(* Logix 5000 Rung export; software revision 16.04 *)

TYPE RLX2_UTIL :   // Internal tag used for internal ladder processing. Not to be updated by user application
STRUCT
   ImgVersionInformation : SINT[28];   // *Do Not Modify*
   RadioInformation : SINT[296];   // *Do Not Modify*
   CRCInformation : DINT[20];   // *Do Not Modify*
   TotalupTime : DINT;   // *Do Not Modify*
   TotalLinkTime : DINT;   // *Do Not Modify*
END_STRUCT
END_TYPE

TYPE RLX2_CONTROL :   // Contains trigger bit for the functions supported by the RLX2. Bit should be set as 1 to trigger AOI request
STRUCT
   GetStatusData : BOOL;   // Reads Diagnostic status data from RLX2
   GetCRCSignature : BOOL;   // Read CRC File Signature Information
END_STRUCT
END_TYPE

TYPE RLX2_STATUS :   // RLX2 Radio Status Data
STRUCT
   SSID : SINT[32];   // The Service Set Identifier is a name assigned to the wireless network
   IPAddress : INT[4];   // Radio's IP address
   MACAddress : SINT[6];   // Physical Media Access Control (MAC) address of the device
   NetworkMode : SINT;   // RLX2 radio Network mode (Master= 6 Repeater=7 Client=1)
   ConnectionState : SINT;   // Connection State of Radio
   SignalStrength : INT;   // Current Strength of the signal in dBm
   Channel : INT;   // Current Channel in which RLX2 is transmitting
   WEP : SINT;   // WEP encryption key
   Flags : DINT;   // Flags: Flag[0/1]= Extension channel Flag[2]= SSIDhidden Flag[3]=Allow Children Flag[4/5]=STP/RSTP Flag[6]=TXusingGI
   MasterMACAddress : SINT[6];   // MAC Address of Parent Radio in which Repeater or Client is linked
   HopCount : SINT;   // Number of hops to the master
   PortStatus : SINT;   // Ethernet Port Status (Speed 1=10Mb/s 2=100Mb/s 3=1000Mb/s)
   Associations : INT;   // Number of network elements to which radio has wireless connection
   BridgeAssociations : INT;   // Number of devices to which radio has wireless connection
   TxRadioThroughput : DINT;   // Transmit throughput in kilobits per second
   RxRadioThroughput : DINT;   // Receive throughput in kilobits per second
   Uptime : RLX2_UPTIME;   // This is the amount of time the radio has been running since power up (Days/Hours/Minutes/Seconds)
   LinkTime : RLX2_LINKTIME;   // The time the radio has been linked (Days/Hours/Minutes/Seconds)
   TxPacketRate : DINT;   // Total number of packets transmitted
   RxPacketRate : DINT;   // Total number of packets received
   ModuleName : SINT[32];   // The name of the radio
   ProductName : SINT[32];   // Name of product family
   ImageVerStr : SINT[28];   // Firmware version loaded in device
   TxGood : DINT;   // Number of Good Transmitted Frames
   RxGood : DINT;   // Number of Good Received Frames
   TxBad : DINT;   // Number of Bad Transmitted Frames
   RxBad : DINT;   // Number of Bad Received Frames
   TxDirectedFrames : DINT;   // Number of Transmitted Directed Frames
   TxMulticastFrames : DINT;   // Number of Transmitted Multicast Frames
   TxBroadcastFrames : DINT;   // Number of Transmitted Broadcast Frames
   RxDirectedFrames : DINT;   // Number of Received Directed Frames
   RxMulticastFrames : DINT;   // Number of Received Multicast Frames
   RxBroadcastFrames : DINT;   // Number of Received Broadcast Frames
   RxCRCErr : DINT;   // Number of CRC Errors
   Retries : SINT;   // Percentage retransmission (0-100%)
   Utilization : SINT;   // Measured channel utilization (0-100%)
   ChannelWidth : SINT;   // Configured channel width (20 or 40 MHz)
   Antennas : SINT;   // Active Antenna Information
   TxRate : INT;   // Encoded Current Tx Rate to Parent (Client/Repeater Only)
   TxBitRate : INT;   // Actual Tx Bit Rate to Parent in 100 kb/s units
   TxBcastRate : INT;   // Broadcast packet rate being sent to radio (pps)
   TxMcstRate : INT;   // Multicast packet rate being sent to radio (pps)
   Reserved1 : DINT;   // Reserved
   Reserved2 : DINT;   // Reserved
   Reserved3 : DINT;   // Reserved
   Reserved4 : DINT;   // Reserved
   Reserved5 : DINT;   // Reserved
   Reserved6 : DINT;   // Reserved
   Reserved7 : DINT;   // Reserved
   Reserved8 : DINT;   // Reserved
   Reserved9 : DINT;   // Reserved
   Reserved10 : DINT;   // Reserved
   Reserved11 : DINT;   // Reserved
   Reserved12 : DINT;   // Reserved
   Reserved13 : DINT;   // Reserved
   Reserved14 : DINT;   // Reserved
   Reserved15 : DINT;   // Reserved
   Reserved16 : DINT;   // Reserved
END_STRUCT
END_TYPE

TYPE RLX2_LINKTIME :   // RLX2 Repeater Link Time
STRUCT
   Days : DINT;   // Number of Days Repeater has been connected with a Master
   Hours : DINT;   // Number of Hours Repeater has been connected with a Master
   Minutes : DINT;   // Number of Minutes Repeater has been connected with a Master
   Seconds : DINT;   // Number of Seconds Repeater has been connected with a Master
END_STRUCT
END_TYPE

TYPE RLX2_UPTIME :
STRUCT
   Days : DINT;
   Hours : DINT;
   Minutes : DINT;
   Seconds : DINT;
END_STRUCT
END_TYPE

TYPE RLX2_CRC :   // CRC File Signature Information
STRUCT
   OS_Sig : DINT;   // CRC signature of OS related files
   Wireless_Sig : DINT;   // CRC signature of Wireless related files
   Config_Sig : DINT;   // CRC signature of Configuration related files
   Security_Sig : DINT;   // CRC signature of Security related files
   Web_Sig : DINT;   // CRC signature of the web pages image file.
   SDCard_Sig : DINT;   // CRC signature of the contents of the SD Card
   Reserved1 : DINT;   // Reserved
   Reserved2 : DINT;   // Reserved
   Reserved3 : DINT;   // Reserved
   Reserved4 : DINT;   // Reserved
   Reserved5 : DINT;   // Reserved
   Reserved6 : DINT;   // Reserved
   Reserved7 : DINT;   // Reserved
   Reserved8 : DINT;   // Reserved
   Reserved9 : DINT;   // Reserved
   Reserved10 : DINT;   // Reserved
   Reserved11 : DINT;   // Reserved
   Reserved12 : DINT;   // Reserved
   Reserved13 : DINT;   // Reserved
   Reserved14 : DINT;   // Reserved
END_STRUCT
END_TYPE

TYPE RLX2_ModuleDef :   // Main RLX2 Radio definition
STRUCT
   CONTROL : RLX2_CONTROL;   // Trigger bits used to request functions from RLX2 Radio
   STATUS : RLX2_STATUS;   // RLX2 radio diagnostic data
   CRC : RLX2_CRC;   // RLX2 CRC file signature Information
   UTIL : RLX2_UTIL;   // *Do Not Modify*
END_STRUCT
END_TYPE

ADD_ON_INSTRUCTION AOI_RLX2   (* revision 2.0, vendor ProSoft Technology Inc., ExecutePrescan *)
// Add-On Instruction for RLX2 Industrial Hotspot
// Revision note:
// 2.0 -- Added Support for Extended Status and CRC File Information (v38)
// Help:
// 1.5 - Fix to Logic to display correct RSSI
// 1.4 --  Change the display information for the Link and Uptime of the radio
VAR_IN_OUT
   RLX2 : RLX2_ModuleDef; {required}
   RLX2_MSG_GET_IMG_VER : MESSAGE; {required}
   RLX2_MSG_GET_STATUS : MESSAGE; {required}
   RLX2_MSG_GET_CRC_SIG : MESSAGE; {required}
END_VAR
VAR
   Hold64 : INT[2];
   HoldRSSI : INT;
   Hold66 : INT[2];
   ImgVersion : DINT;
   TriggerStatusMSG : BOOL;   // Trigger Status Information MSG
END_VAR

ROUTINE Logic   (* ladder *)
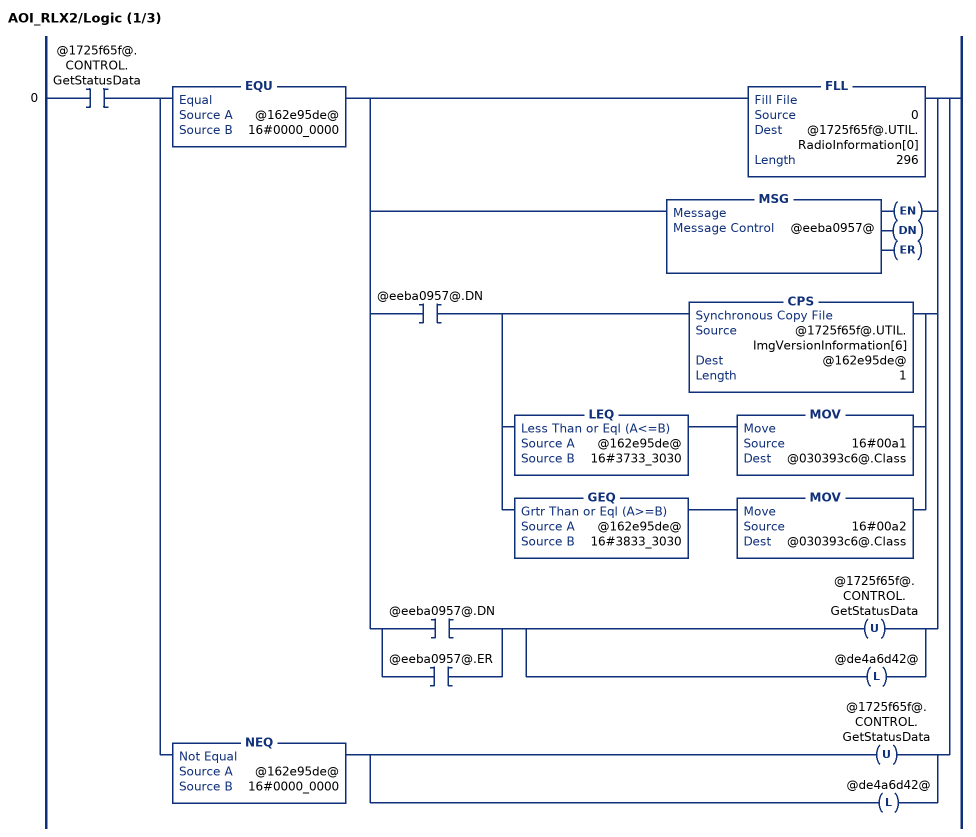
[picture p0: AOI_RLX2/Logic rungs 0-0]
   0: XIC(@1725f65f@.CONTROL.GetStatusData)[EQU(@162e95de@,16#0000_0000) [FLL(0,@1725f65f@.UTIL.RadioInformation[0],296) ,MSG(@eeba0957@) ,[XIC(@eeba0957@.DN) [CPS(@1725f65f@.UTIL.ImgVersionInformation[6],@162e95de@,1) ,LEQ(@162e95de@,16#3733_3030) MOV(16#00a1,@030393c6@.Class) ,GEQ(@162e95de@,16#3833_3030) MOV(16#00a2,@030393c6@.Class) ] ,[XIC(@eeba0957@.DN) ,XIC(@eeba0957@.ER) ] [OTU(@1725f65f@.CONTROL.GetStatusData) ,OTL(@de4a6d42@) ] ] ] ,NEQ(@162e95de@,16#0000_0000) [OTU(@1725f65f@.CONTROL.GetStatusData) ,OTL(@de4a6d42@) ] ];
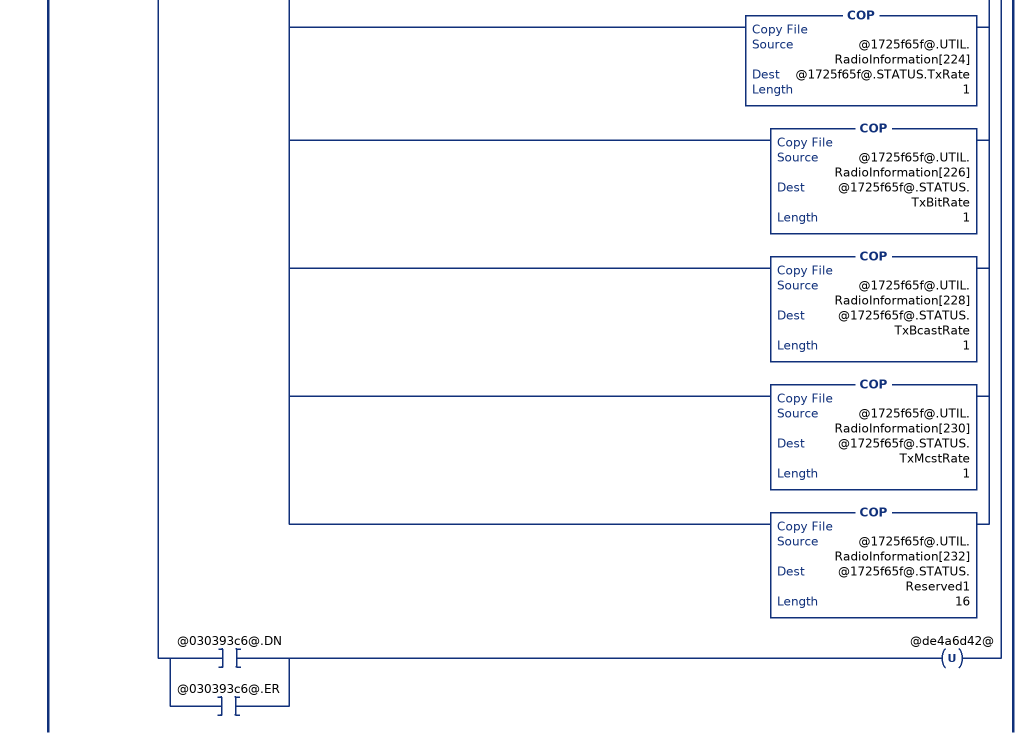
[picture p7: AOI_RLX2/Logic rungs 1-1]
   1: XIC(@de4a6d42@)[MSG(@030393c6@) ,[XIC(@030393c6@.DN) [COP(@1725f65f@.UTIL.RadioInformation[0],@1725f65f@.STATUS.SSID[0],32) ,MVM(@1725f65f@.UTIL.RadioInformation[32],255,@1725f65f@.STATUS.IPAddress[0]) ,MVM(@1725f65f@.UTIL.RadioInformation[33],255,@1725f65f@.STATUS.IPAddress[1]) ,MVM(@1725f65f@.UTIL.RadioInformation[34],255,@1725f65f@.STATUS.IPAddress[2]) ,MVM(@1725f65f@.UTIL.RadioInformation[35],255,@1725f65f@.STATUS.IPAddress[3]) ,COP(@1725f65f@.UTIL.RadioInformation[36],@1725f65f@.STATUS.MACAddress[0],6) ,COP(@1725f65f@.UTIL.RadioInformation[42],@1725f65f@.STATUS.NetworkMode,1) ,COP(@1725f65f@.UTIL.RadioInformation[43],@1725f65f@.STATUS.ConnectionState,1) ,NEQ(@1725f65f@.STATUS.NetworkMode,6) COP(@1725f65f@.UTIL.RadioInformation[44],@0dfc57aa@,1) SUB(@0dfc57aa@,100,@1725f65f@.STATUS.SignalStrength) ,MVM(@1725f65f@.UTIL.RadioInformation[46],255,@1725f65f@.STATUS.Channel) ,COP(@1725f65f@.UTIL.RadioInformation[47],@1725f65f@.STATUS.WEP,1) ,COP(@1725f65f@.UTIL.RadioInformation[48],@1725f65f@.STATUS.Flags,4) ,COP(@1725f65f@.UTIL.RadioInformation[52],@1725f65f@.STATUS.MasterMACAddress[0],6) ,COP(@1725f65f@.UTIL.RadioInformation[58],@1725f65f@.STATUS.HopCount,1) ,COP(@1725f65f@.UTIL.RadioInformation[59],@1725f65f@.STATUS.PortStatus,1) ,COP(@1725f65f@.UTIL.RadioInformation[60],@1725f65f@.STATUS.Associations,2) ,COP(@1725f65f@.UTIL.RadioInformation[62],@1725f65f@.STATUS.BridgeAssociations,2) ,COP(@1725f65f@.UTIL.RadioInformation[64],@dc9c6250@[0],1) COP(@dc9c6250@[0],@1725f65f@.STATUS.TxRadioThroughput,1) ,COP(@1725f65f@.UTIL.RadioInformation[66],@0cd69a93@[0],1) COP(@0cd69a93@[0],@1725f65f@.STATUS.RxRadioThroughput,1) ,[COP(@1725f65f@.UTIL.RadioInformation[68],@1725f65f@.UTIL.TotalupTime,4) ,CPT(@1725f65f@.STATUS.Uptime.Days,(@1725f65f@.UTIL.TotalupTime/60/60/24)) ,CPT(@1725f65f@.STATUS.Uptime.Hours,(@1725f65f@.UTIL.TotalupTime/60/60)-(@1725f65f@.STATUS.Uptime.Days*24)) ,CPT(@1725f65f@.STATUS.Uptime.Minutes,(@1725f65f@.UTIL.TotalupTime/60)-(@1725f65f@.STATUS.Uptime.Days*24*60)-(@1725f65f@.STATUS.Uptime.Hours*60)) ,CPT(@1725f65f@.STATUS.Uptime.Seconds,(@1725f65f@.UTIL.TotalupTime)-(@1725f65f@.STATUS.Uptime.Days*24*60*60)-(@1725f65f@.STATUS.Uptime.Hours*60*60)-(@1725f65f@.STATUS.Uptime.Minutes*60)) ] ,[COP(@1725f65f@.UTIL.RadioInformation[72],@1725f65f@.UTIL.TotalLinkTime,4) ,CPT(@1725f65f@.STATUS.LinkTime.Days,(@1725f65f@.UTIL.TotalLinkTime/60/60/24)) ,CPT(@1725f65f@.STATUS.LinkTime.Hours,(@1725f65f@.UTIL.TotalLinkTime/60/60)-(@1725f65f@.STATUS.LinkTime.Days*24)) ,CPT(@1725f65f@.STATUS.LinkTime.Minutes,(@1725f65f@.UTIL.TotalLinkTime/60)-(@1725f65f@.STATUS.LinkTime.Days*24*60)-(@1725f65f@.STATUS.LinkTime.Hours*60)) ,CPT(@1725f65f@.STATUS.LinkTime.Seconds,(@1725f65f@.UTIL.TotalLinkTime)-(@1725f65f@.STATUS.LinkTime.Days*24*60*60)-(@1725f65f@.STATUS.LinkTime.Hours*60*60)-(@1725f65f@.STATUS.LinkTime.Minutes*60)) ] ,COP(@1725f65f@.UTIL.RadioInformation[76],@1725f65f@.STATUS.TxPacketRate,4) ,COP(@1725f65f@.UTIL.RadioInformation[80],@1725f65f@.STATUS.RxPacketRate,4) ,COP(@1725f65f@.UTIL.RadioInformation[84],@1725f65f@.STATUS.ModuleName[0],32) ,COP(@1725f65f@.UTIL.RadioInformation[116],@1725f65f@.STATUS.ProductName[0],32) ,COP(@1725f65f@.UTIL.RadioInformation[148],@1725f65f@.STATUS.ImageVerStr[0],28) ,COP(@1725f65f@.UTIL.RadioInformation[176],@1725f65f@.STATUS.TxGood,4) ,COP(@1725f65f@.UTIL.RadioInformation[180],@1725f65f@.STATUS.RxGood,4) ,COP(@1725f65f@.UTIL.RadioInformation[184],@1725f65f@.STATUS.TxBad,4) ,COP(@1725f65f@.UTIL.RadioInformation[188],@1725f65f@.STATUS.RxBad,4) ,COP(@1725f65f@.UTIL.RadioInformation[192],@1725f65f@.STATUS.TxDirectedFrames,4) ,COP(@1725f65f@.UTIL.RadioInformation[196],@1725f65f@.STATUS.TxMulticastFrames,4) ,COP(@1725f65f@.UTIL.RadioInformation[200],@1725f65f@.STATUS.TxBroadcastFrames,4) ,COP(@1725f65f@.UTIL.RadioInformation[204],@1725f65f@.STATUS.RxDirectedFrames,4) ,COP(@1725f65f@.UTIL.RadioInformation[208],@1725f65f@.STATUS.RxMulticastFrames,4) ,COP(@1725f65f@.UTIL.RadioInformation[212],@1725f65f@.STATUS.RxBroadcastFrames,4) ,COP(@1725f65f@.UTIL.RadioInformation[216],@1725f65f@.STATUS.RxCRCErr,4) ,COP(@1725f65f@.UTIL.RadioInformation[220],@1725f65f@.STATUS.Retries,1) ,COP(@1725f65f@.UTIL.RadioInformation[221],@1725f65f@.STATUS.Utilization,1) ,COP(@1725f65f@.UTIL.RadioInformation[222],@1725f65f@.STATUS.ChannelWidth,1) ,COP(@1725f65f@.UTIL.RadioInformation[223],@1725f65f@.STATUS.Antennas,1) ,COP(@1725f65f@.UTIL.RadioInformation[224],@1725f65f@.STATUS.TxRate,1) ,COP(@1725f65f@.UTIL.RadioInformation[226],@1725f65f@.STATUS.TxBitRate,1) ,COP(@1725f65f@.UTIL.RadioInformation[228],@1725f65f@.STATUS.TxBcastRate,1) ,COP(@1725f65f@.UTIL.RadioInformation[230],@1725f65f@.STATUS.TxMcstRate,1) ,COP(@1725f65f@.UTIL.RadioInformation[232],@1725f65f@.STATUS.Reserved1,16) ] ,[XIC(@030393c6@.DN) ,XIC(@030393c6@.ER) ] OTU(@de4a6d42@) ] ];
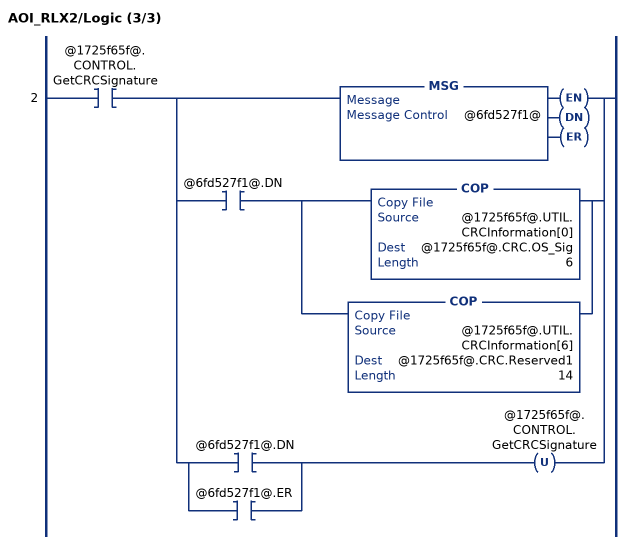
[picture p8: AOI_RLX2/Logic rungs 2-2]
   2: XIC(@1725f65f@.CONTROL.GetCRCSignature)[MSG(@6fd527f1@) ,[XIC(@6fd527f1@.DN) [COP(@1725f65f@.UTIL.CRCInformation[0],@1725f65f@.CRC.OS_Sig,6) ,COP(@1725f65f@.UTIL.CRCInformation[6],@1725f65f@.CRC.Reserved1,14) ] ,[XIC(@6fd527f1@.DN) ,XIC(@6fd527f1@.ER) ] OTU(@1725f65f@.CONTROL.GetCRCSignature) ] ];
END_ROUTINE

ROUTINE Prescan   (* ladder *)
// Reset ImgVersion on PLC transitions from PROGRAM -> RUN mode or powers up
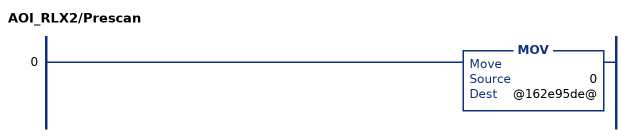
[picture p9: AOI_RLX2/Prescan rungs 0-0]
   0: MOV(0,@162e95de@);
END_ROUTINE
END_ADD_ON_INSTRUCTION

VAR_GLOBAL   (* controller tags *)
   RLX2 : RLX2_ModuleDef;
   AOI_RLX2 : AOI_RLX2;
   RLX2_MSGgetStatus : MESSAGE;
        MessageParameters(MessageType := CIP Generic, ConnectedFlag := 2, ConnectionPath := RLX2, ServiceCode := 16#0001, ObjectType := 16#00a2, TargetObject := 1, LocalElement := RLX2.UTIL.RadioInformation[0], DestinationTag := RLX2.UTIL.RadioInformation[0])
   RLX2_MSGgetImgVers : MESSAGE;
        MessageParameters(MessageType := CIP Generic, ConnectedFlag := 2, ConnectionPath := RLX2, ServiceCode := 16#000e, ObjectType := 16#00a1, TargetObject := 1, AttributeNumber := 16#0017, DestinationTag := RLX2.UTIL.ImgVersionInformation)
   RLX2_MSGgetCRC : MESSAGE;
        MessageParameters(MessageType := CIP Generic, ConnectedFlag := 2, ConnectionPath := RLX2, ServiceCode := 16#0001, ObjectType := 16#00a3, TargetObject := 1, LocalElement := RLX2.UTIL.CRCInformation[0], DestinationTag := RLX2.UTIL.CRCInformation[0])
END_VAR

PROGRAM MainProgram

ROUTINE MainRoutine   (* ladder *)
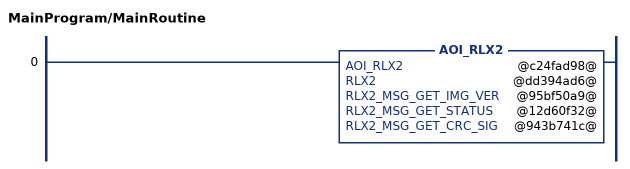
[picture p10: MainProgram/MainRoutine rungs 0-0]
   0: AOI_RLX2(@c24fad98@,@dd394ad6@,@95bf50a9@,@12d60f32@,@943b741c@);
END_ROUTINE
END_PROGRAM
